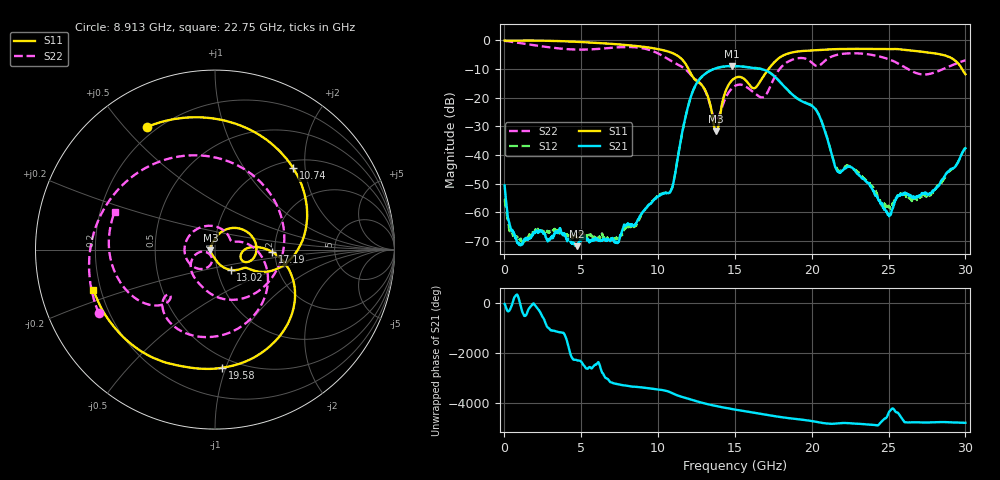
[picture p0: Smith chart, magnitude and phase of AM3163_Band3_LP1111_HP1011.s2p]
!Agilent Technologies,E8364B,MY43040894,A.07.50.67
!Agilent E8364B: A.07.50.67
!Date: Thursday, August 20, 2020 12:18:08
!Correction: S11(Full 2 Port(1,2))
!S21(Full 2 Port(1,2))
!S12(Full 2 Port(1,2))
!S22(Full 2 Port(1,2))
!S2P File: Measurements: S11, S21, S12, S22:
# Hz S  dB  R 50
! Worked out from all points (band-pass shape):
!   3201 points, 10 MHz to 30 GHz, reference 50 ohm
!   highest |S21| = -8.92 dB at 14.79 GHz (marker M1); lowest = -71.8 dB at 4.733 GHz (marker M2)
!   |S21| within 3 dB of the highest: 13 GHz to 17.44 GHz (4.437 GHz wide, 29.2 % of centre)
!   lowest |S11| = -31.7 dB at 13.78 GHz (marker M3), VSWR 1.05, Z = 47.5 - j0.303 ohm
!   |S11| at or under -10 dB: 11.98 GHz to 17.18 GHz (5.201 GHz wide, 35.7 % of centre); 29.78 GHz to end of sweep
!   |S22| runs from -28.0 to -0.2 dB; largest |S21 - S12| = 0.0098
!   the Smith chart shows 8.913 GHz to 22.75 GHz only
!   S11 on the Smith chart (normalised r, x): 8.913 GHz: 0.16, +0.58; 10.74 GHz: 1.15, +1.73; 13.02 GHz: 1.16, -0.27; 17.19 GHz: 1.93, -0.05; 19.58 GHz: 0.42, -0.97; 22.75 GHz: 0.17, -0.16
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1e7  -0.06 -2.1  -50.63 -57.7  -55.39 26.9  -0.16 -4.8
1.228344e9  -0.01 -33.1  -70.55 -107.9  -70.30 -24.2  -1.10 -81.0
2.596638e9  -0.09 -69.7  -67.58 23.3  -67.03 -148.8  -2.17 -159.0
4.733425e9  -0.49 -125.2  -71.83 -152.2  -68.85 -163.3  -3.18 89.0
5.014581e9  -0.56 -132.4  -69.56 138.8  -68.11 -61.4  -3.21 74.0
6.720262e9  -1.10 -176.8  -69.37 -174.9  -68.96 38.7  -2.67 -20.3
7.882375e9  -1.59 150.8  -64.44 -76.2  -65.42 -85.4  -2.28 -87.2
8.913281e9  -2.14 118.9  -60.52 -149.3  -60.71 -151.6  -2.64 -151.2
1.000979e10  -3.02 78.8  -54.47 129.6  -54.23 128.4  -4.57 127.5
1.07408e10  -4.02 46.3  -53.17 29.0  -53.05 31.3  -6.80 58.2
1.301816e10  -16.93 -52.5  -11.84 -69.6  -11.86 -68.7  -17.06 -156.3
1.377728e10  -31.70 -172.9  -9.69 -174.7  -9.69 -174.7  -27.95 -135.5
1.478945e10  -14.03 31.8  -8.92 66.5  -9.06 67.4  -16.81 -133.4
1.5005e10  -13.10 17.6  -8.94 43.5  -9.05 44.7  -15.89 -150.2
1.718865e10  -9.97 -2.2  -10.98 -178.4  -10.93 -177.7  -17.40 19.2
1.957848e10  -3.61 -86.5  -21.79 -16.3  -21.69 -15.5  -6.32 -119.1
2.000958e10  -3.49 -98.2  -22.82 -55.5  -22.66 -55.1  -7.79 -135.4
2.164966e10  -3.02 -137.1  -45.52 -149.3  -44.91 -145.8  -5.03 -161.9
2.274617e10  -2.93 -161.6  -45.06 -154.6  -45.10 -155.8  -4.47 159.3
2.500479e10  -3.04 145.3  -60.95 -77.0  -58.03 173.8  -6.55 67.9
2.740399e10  -4.10 77.9  -53.25 -111.1  -53.92 -117.6  -11.90 -88.2
3e10  -11.76 -28.3  -37.64 -126.0  -37.42 -124.5  -6.96 130.5
